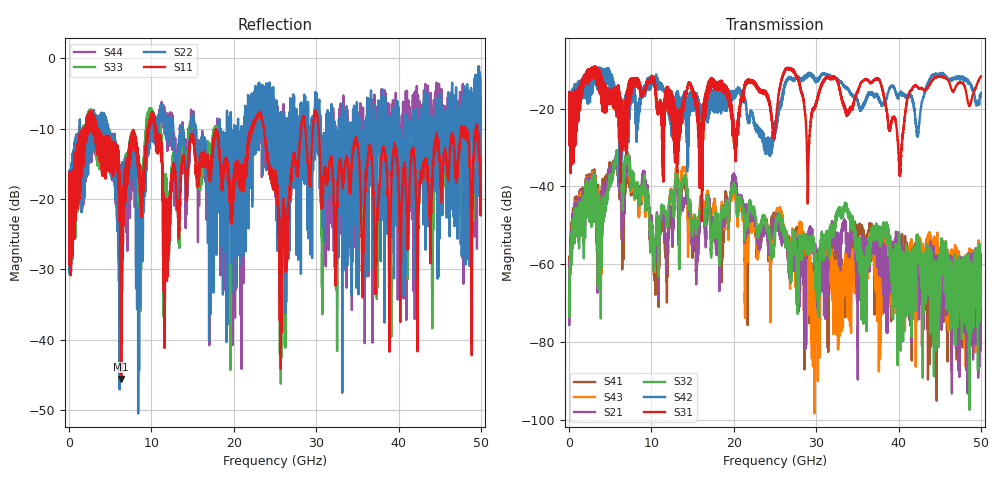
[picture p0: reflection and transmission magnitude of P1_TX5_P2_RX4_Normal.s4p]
!Keysight Technologies,N5225B,MY57041031,A.13.20.10
!Date: Friday, May 31, 2019 11:33:37
!Correction: S11(Full 4 Port(1,2,3,4))
!S12(Full 4 Port(1,2,3,4))
!S13(Full 4 Port(1,2,3,4))
!S14(Full 4 Port(1,2,3,4))
!S21(Full 4 Port(1,2,3,4))
!S22(Full 4 Port(1,2,3,4))
!S23(Full 4 Port(1,2,3,4))
!S24(Full 4 Port(1,2,3,4))
!S31(Full 4 Port(1,2,3,4))
!S32(Full 4 Port(1,2,3,4))
!S33(Full 4 Port(1,2,3,4))
!S34(Full 4 Port(1,2,3,4))
!S41(Full 4 Port(1,2,3,4))
!S42(Full 4 Port(1,2,3,4))
!S43(Full 4 Port(1,2,3,4))
!S44(Full 4 Port(1,2,3,4))
!S4P File: Measurements: <S11,S12,S13,S14>,
!<S21,S22,S23,S24>,
!<S31,S32,S33,S34>,
!<S41,S42,S43,S44>:
# Hz S  dB  R 50.0
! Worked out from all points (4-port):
!   5000 points, 10 MHz to 50 GHz, reference 50 ohm
!   strongest paths, dB at 10 MHz, 12.51 GHz, 25.01 GHz, 37.51 GHz, 50 GHz:
!     S31: -19.3, -23.1, -26.1, -12.3, -11.7
!     S42: -19.6, -27.3, -24.0, -17.0, -16.0
!     S32: -73.5, -42.7, -52.8, -50.3, -67.6
!     S21: -68.2, -52.7, -49.2, -56.5, -67.3
!     S43: -75.4, -42.1, -50.1, -61.4, -60.9
!     S41: -58.1, -52.4, -47.5, -57.1, -62.3
!   lowest |S11| = -45.6 dB at 6.34 GHz (marker M1), VSWR 1.01, Z = 49.6 - j0.303 ohm
!   |S11| at or under -10 dB: 3.502 GHz to 9.556 GHz (6.054 GHz wide, 92.7 % of centre); 10.5 GHz to 22.11 GHz (11.6 GHz wide, 71.2 % of centre); 30.29 GHz to 47.6 GHz (17.31 GHz wide, 44.4 % of centre)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
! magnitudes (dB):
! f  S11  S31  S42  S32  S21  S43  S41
! 10 MHz  -19.7  -19.3  -19.6  -73.5  -68.2  -75.4  -58.1
! 720 MHz  -22.3  -20.4  -19.5  -45.7  -44.2  -44.1  -42.8
! 6.34 GHz  -45.6  -20.2  -26.2  -34.1  -36.7  -35.5  -38.9
! 10.34 GHz  -8.7  -13.1  -11.9  -59.9  -57.7  -62.1  -64.1
! 37.45 GHz  -22.8  -12.2  -17.0  -50.7  -56.3  -71.2  -59.8
! 40.18 GHz  -26.2  -37.3  -16.0  -65.1  -56.1  -66.1  -57.1
! 50 GHz  -18.2  -11.7  -16.0  -67.6  -67.3  -60.9  -62.3
